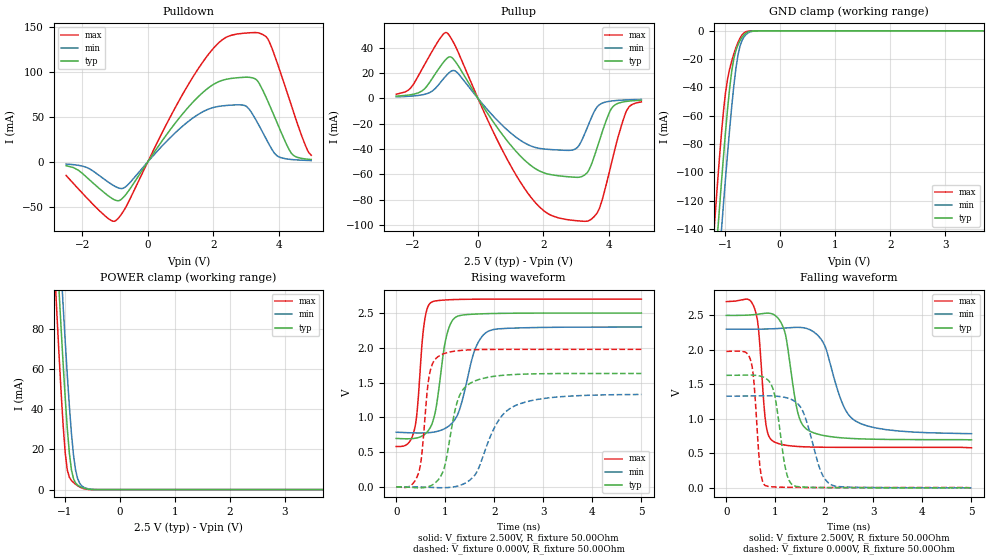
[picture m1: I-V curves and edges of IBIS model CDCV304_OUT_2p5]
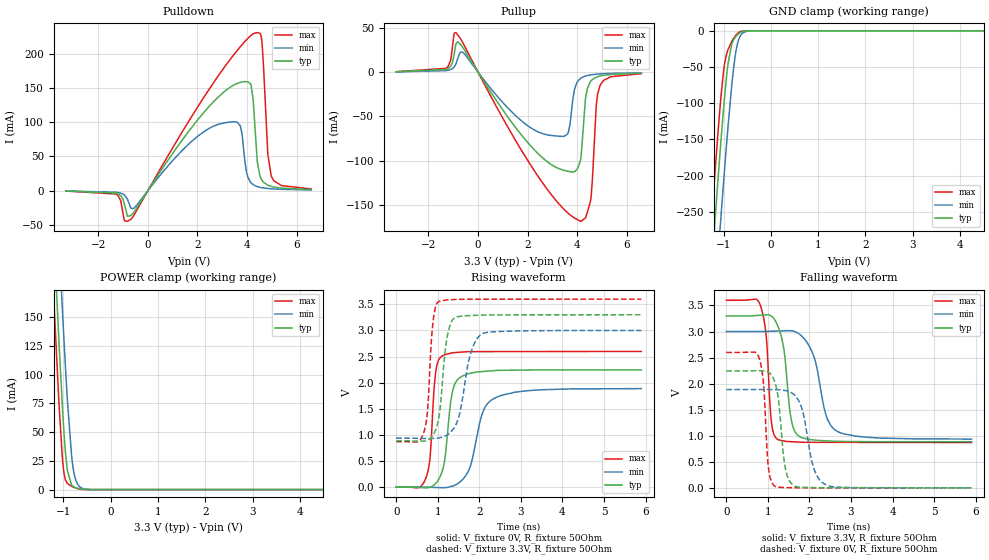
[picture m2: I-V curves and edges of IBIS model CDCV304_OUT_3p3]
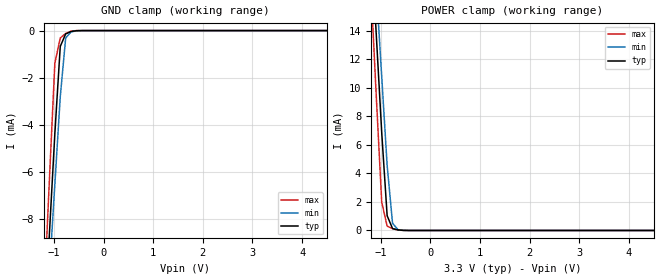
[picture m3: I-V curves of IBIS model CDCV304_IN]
|Texas Instruments Incorporated
|200-MHz General Purpose Clock Buffer, PCI-X Compliant
| Marketing part#   Voltage Range   Package-type   #pins
|CDCV304PW   2.3V - 3.6V   TSSOP   8-pin PW
|CDCV304PWG4   2.3V - 3.6V   TSSOP   8-pin PW
|CDCV304PWR   2.3V - 3.6V   TSSOP   8-pin PW
|CDCV304PWRG4   2.3V - 3.6V   TSSOP   8-pin PW
[IBIS Ver]   4.0
[File name]   cdcv304.ibs
[File Rev]   1.3
[Date]   01/30/2015
[Source]   Texas Instruments Incorporated.
   Analog-eLab, HPA
   12500 TI Blvd
   Dallas, TX -75243
   For Support e-mail: elab_ibis@list.ti.com
[Notes]   Revision History:
   Rev 1.1: 11/15/2009
   - Covers industrial temp range
   - All test data contained in this file are derived from
   hspice(tm) simulations.
   - File created by CDC Systems and Application
   Rev 1.2: 07/03/2009
   - Added CDCV304_OUT_2p5 model for 2.5V supply
   - CDCV304_OUT_2p5 model generated from TISPICED simulations
   - Non-monotonic warnings relay true buffer behavior for pullup/down
   - Added [Model Selector] to choose between 2.5V or 3.3V model.
   - Ccomp values are based on simulation setup in TISPICED,
   part uses BJT devices.
   Rev 1.3: 01/30/2015
   - Updated CDCV304_OUT_3p3 model from TISPICED simulations
   - Non-monotonic warnings relay true buffer behavior for pullup/down
[Disclaimer]
 This product is designed as an aid for customers of Texas Instruments.
 No warranties, either expressed or implied, with respect to this third
 party software (if any) or with respect to its fitness for any
 particular purpose is claimed by Texas Instruments or the author. The
 software (if any) is provided solely on an "as is" basis. The entire
 risk as to its quality and performance is with the customer
[Copyright] (C) Copyright 2009 Texas Instruments Incorporated.
   All rights reserved.
|   CDCV304PW Component
[Component]   CDCV304PW
[Manufacturer]  Texas Instruments, Inc.
[Package]   |8-pin PW TSSOP package,
|   typ   min   max
R_pkg   0.040   0.034   0.046
L_pkg   2.625nH   2.419nH   2.861nH
C_pkg   0.304pF   0.286pF   0.321pF
[Pin]   signal_name   model_name   R_pin   L_pin   C_pin
1   CLKIN   CDCV304_IN   0.12421  3.18009nH  0.51182pF
2   OE   CDCV304_IN   0.12681  2.66769nH  0.47449pF
3   1Y0   CDCV304_OUT   0.13711  2.77393nH  0.48053pF
4   GND   GND   0.08098  3.03663nH  0.54744pF
5   1Y1   CDCV304_OUT   0.12638  3.20754nH  0.51379pF
6   VDD   POWER   0.07180  2.38222nH  0.49957pF
7   1Y2   CDCV304_OUT   0.14173  2.82266nH  0.48353pF
8   1Y3   CDCV304_OUT   0.12849  3.22359nH  0.51572pF
[Model Selector] CDCV304_OUT
CDCV304_OUT_2p5   2.5V Tristate Output
CDCV304_OUT_3p3   3.3V Tristate Output
| Models and submodels in the file (3): CDCV304_OUT_2p5 (3-state), CDCV304_OUT_3p3 (3-state), CDCV304_IN (Input)
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|   Model CDCV304_OUT_2p5
[Model]   CDCV304_OUT_2p5
Model_type   3-state
Polarity   Non-Inverting
Enable   Active-High
Vmeas = 1.25V   |Vref for timing measurements.
Cref = 25pF   |load capacitance for timing spec.
Rref = 500   |500 Ohm to GND.
Vref = 0   |Timing specification test load voltage; GND
|   typ   min   max
C_comp   2.454pF   2.480pF   2.429pF
[Temperature range]   27   85   -40
[Voltage range]   2.5   2.3   2.7
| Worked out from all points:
|   slope of the pulldown table from 0 to 0.375 V, typ, clamps not added: 18.7 ohm
|   slope of the pullup table from 0 to 0.375 V, typ, clamps not added: 25.1 ohm
|   GND clamp passes 1 mA (typ) near -0.59 V on its own axis
|   POWER clamp passes 1 mA (typ) near -0.68 V on its own axis
|   falling waveform, V_fixture 2.500V, R_fixture 50.00Ohm: 20-80 % time 242ps typ, 425ps min, 133ps max; typ from 2.5 V to 0.696 V
|   rising waveform, V_fixture 2.500V, R_fixture 50.00Ohm: 20-80 % time 225ps typ, 339ps min, 143ps max; typ from 0.696 V to 2.5 V
|   rising waveform, V_fixture 0.000V, R_fixture 50.00Ohm: 20-80 % time 287ps typ, 529ps min, 159ps max; typ from 0 V to 1.63 V
|   falling waveform, V_fixture 0.000V, R_fixture 50.00Ohm: 20-80 % time 197ps typ, 325ps min, 117ps max; typ from 1.63 V to 0 V
[Pulldown]
|   Voltage   I(typ)   I(min)   I(max)
-2.5V     -4.282mA   -2.476mA   -15.1mA
-992.5mV  -42.64mA   -27.45mA   -65.62mA
-653.3mV  -35.48mA   -26.93mA   -49.07mA
703.5mV   36.48mA    27.44mA    50.95mA
1.683V    76.98mA    55.58mA    110.8mA
2.324V    90.93mA    62.24mA    136.6mA
2.965V    93.85mA    62.47mA    142.8mA
3.342V    90.38mA    44.32mA    143.3mA
3.681V    66.49mA    21.35mA    135.8mA
3.945V    44.26mA    6.972mA    111.2mA
4.397V    9.233mA    2.555mA    62.09mA
5V        2.556mA    1.432mA    7.256mA
[GND Clamp]
|   Voltage   I(typ)   I(min)   I(max)
-2.5V     -918mA     -929.6mA   -913.4mA
-1.219V   -187mA     -219.9mA   -151.3mA
-1.181V   -166.8mA   -200mA     -130.7mA
-1.143V   -146.8mA   -180.3mA   -110.7mA
-1.106V   -127.2mA   -160.9mA   -91.4mA
-1.068V   -108mA     -141.7mA   -73.33mA
-992.5mV  -71.68mA   -104.5mA   -43.83mA
-879.4mV  -28.61mA   -53.58mA   -21.34mA
-766.3mV  -9.997mA   -17.27mA   -8.262mA
-691mV    -4.522mA   -6.7mA     -2.852mA
-615.6mV  -1.453mA   -2.46mA    -549.6uA
5V        0A         0A         0A
[Pullup]
|   Voltage   I(typ)   I(min)   I(max)
-2.5V     1.763mA    1.188mA    3.233mA
-1.709V   5.877mA    2.781mA    23.11mA
-954.8mV  31.36mA    18.36mA    51.83mA
-653.3mV  27.69mA    20.84mA    39.24mA
590.5mV   -22.98mA   -17.26mA   -32.81mA
1.533V    -51.12mA   -36.53mA   -74.94mA
2.889V    -62.08mA   -40.79mA   -96.14mA
3.266V    -60.43mA   -27.98mA   -96.94mA
3.719V    -33.2mA    -4.961mA   -86.65mA
4.095V    -7.629mA   -2.04mA    -50.06mA
4.548V    -2.38mA    -1.199mA   -9.673mA
5V        -1.438mA   -849uA     -2.733mA
[POWER Clamp]
|   Voltage   I(typ)   I(min)   I(max)
-2.5V     889.6mA    895.1mA    893.4mA
-1.181V   138.6mA    167mA      107.6mA
-1.143V   118.8mA    147.5mA    87.11mA
-1.106V   99.34mA    128.4mA    67.36mA
-1.068V   80.46mA    109.6mA    48.67mA
-1.03V    62.35mA    91.33mA    31.79mA
-992.5mV  45.4mA     73.67mA    18.16mA
-954.8mV  30.26mA    56.9mA     9.72mA
-879.4mV  9.747mA    27.82mA    4.528mA
-804mV    3.293mA    9.602mA    2.651mA
-691mV    1.081mA    1.815mA    792uA
5V        0A         0A         0A
[Ramp]
R_load = 50.00Ohm
|   typ   min   max
dV/dt_r   978.461mV/286.786ps 797.286mV/528.521ps   1.187V/158.780ps
dV/dt_f   1.083V/241.882ps 909.137mV/423.978ps   1.272V/133.440ps
[Falling Waveform]
V_fixture = 2.500V
V_fixture_min = 2.300V
V_fixture_max = 2.700V
R_fixture = 50.00Ohm
|   Time   V(typ)   V(min)   V(max)
0s        2.5V       2.3V       2.7V
580ps     2.512V     2.3V       2.591V
660ps     2.519V     2.3V       2.273V
810ps     2.532V     2.303V     910.5mV
960ps     2.515V     2.306V     672.5mV
1.18ns    2.289V     2.315V     621.3mV
1.45ns    1.112V     2.326V     599.4mV
1.65ns    843.6mV    2.308V     592.7mV
2.64ns    712.2mV    965.7mV    586.2mV
5ns       695.5mV    784.7mV    580.2mV
[Rising Waveform]
V_fixture = 2.500V
V_fixture_min = 2.300V
V_fixture_max = 2.700V
R_fixture = 50.00Ohm
|   Time   V(typ)   V(min)   V(max)
0s        695.5mV    784.7mV    580.2mV
370ps     696.7mV    775.5mV    817.8mV
430ps     704.5mV    774.6mV    1.11V
570ps     749.8mV    775.4mV    2.345V
720ps     888mV      782.8mV    2.657V
1.02ns    2.152V     849.5mV    2.689V
1.23ns    2.448V     1.007V     2.695V
1.61ns    2.485V     1.983V     2.699V
1.9ns     2.492V     2.246V     2.7V
5ns       2.5V       2.3V       2.7V
[Rising Waveform]
V_fixture = 0.000V
V_fixture_min = 0.000V
V_fixture_max = 0.000V
R_fixture = 50.00Ohm
|   Time   V(typ)   V(min)   V(max)
0s        12.14uV    15.12uV    9.328uV
450ps     -14.68mV   -2.158mV   188.3mV
520ps     -14.55mV   -3.527mV   450.7mV
680ps     7.63mV     -7.739mV   1.623V
890ps     131.9mV    -13.27mV   1.889V
1.26ns    1.257V     12.05mV    1.958V
1.57ns    1.512V     140.2mV    1.972V
2.05ns    1.595V     911.9mV    1.977V
2.43ns    1.616V     1.169V     1.978V
5ns       1.631V     1.329V     1.978V
[Falling Waveform]
V_fixture = 0.000V
V_fixture_min = 0.000V
V_fixture_max = 0.000V
R_fixture = 50.00Ohm
|   Time   V(typ)   V(min)   V(max)
0s        1.631V     1.329V     1.978V
500ps     1.634V     1.332V     1.839V
560ps     1.632V     1.332V     1.553V
690ps     1.62V      1.334V     283.6mV
800ps     1.59V      1.334V     29.84mV
960ps     1.416V     1.331V     12.9mV
1.21ns    265.6mV    1.308V     7.152mV
1.37ns    32.08mV    1.265V     5.737mV
2.14ns    1.676mV    43.86mV    3.752mV
5ns       12.14uV    15.12uV    9.328uV
|   Model CDCV304_OUT_3p3
[Model]   CDCV304_OUT_3p3
Model_type   3-state
Polarity   Non-Inverting
Enable   Active-High
Vmeas = 1.5V   |Vref for timing measurements.
Cref = 15pF   |load capacitance for timing spec.
Rref = 50   |500 Ohm to GND.
Vref = 3.3   |Timing specification test load voltage; GND
|   typ   min   max
C_comp   2.8p   1.8p   3.8p
[Voltage Range]   3.3   3   3.6
[Temperature Range]   27   125   -40
[Pullup Reference]   3.3   3   3.6
[Pulldown Reference]   -0   -0   -0
[Power Clamp Reference]   3.3   3   3.6
[GND Clamp Reference]   -0   -0   -0
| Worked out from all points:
|   slope of the pulldown table from 0 to 0.495 V, typ, clamps not added: 18 ohm
|   slope of the pullup table from 0 to 0.495 V, typ, clamps not added: 22.8 ohm
|   GND clamp passes 1 mA (typ) near -0.60 V on its own axis
|   POWER clamp passes 1 mA (typ) near -0.68 V on its own axis
|   falling waveform, V_fixture 3.3V, R_fixture 50Ohm: 20-80 % time 202ps typ, 346ps min, 127ps max; typ from 3.3 V to 0.885 V
|   rising waveform, V_fixture 0V, R_fixture 50Ohm: 20-80 % time 193ps typ, 352ps min, 126ps max; typ from 0 V to 2.24 V
|   rising waveform, V_fixture 3.3V, R_fixture 50Ohm: 20-80 % time 181ps typ, 296ps min, 123ps max; typ from 0.885 V to 3.3 V
|   falling waveform, V_fixture 0V, R_fixture 50Ohm: 20-80 % time 170ps typ, 279ps min, 112ps max; typ from 2.24 V to 0 V
[Pulldown]
|   Voltage   I(typ)   I(min)   I(max)
-3.3V     -532.5uA   -429.4uA   -548.2uA
-1.29V    -3.619mA   -2.276mA   -4.881mA
-943.8mV  -19.98mA   -6.381mA   -43.94mA
-686.4mV  -36.25mA   -25.57mA   -41.88mA
1.947V    100.5mA    77.49mA    118.6mA
3.58V     156.1mA    100.2mA    203.6mA
4.165V    153.9mA    11.37mA    226.7mA
4.412V    42.4mA     6.001mA    230.7mA
4.6V      15.27mA    4.355mA    217.2mA
4.838V    8.061mA    3.213mA    53.29mA
4.976V    6.283mA    2.78mA     21.43mA
6.59V     1.714mA    1.059mA    2.521mA
[GND Clamp]
|   Voltage   I(typ)   I(min)   I(max)
-3.3V     -2.322A    -2.423A    -2.26A
-1.29V    -362.4mA   -471.1mA   -294.8mA
-1.241V   -316.7mA   -425.2mA   -249.3mA
-1.211V   -289.6mA   -397.9mA   -222.4mA
-1.063V   -158.8mA   -264.2mA   -97.15mA
-983.4mV  -95.72mA   -196mA     -48.09mA
-904.2mV  -44.97mA   -131.7mA   -25.96mA
-825mV    -18.13mA   -74.61mA   -14.72mA
-765.6mV  -10.19mA   -40.47mA   -8.301mA
-646.8mV  -2.468mA   -7.184mA   -1.172mA
-409.2mV  -10.16uA   -109.2uA   -598.7nA
6.59V     0A         0A         0A
[Pullup]
|   Voltage   I(typ)   I(min)   I(max)
-3.3V     386.2uA    255uA      448.8uA
-1.29V    3.008mA    1.667mA    4.286mA
-894.3mV  31.44mA    9.002mA    44.56mA
-597.3mV  27.08mA    21.95mA    32.33mA
3.056V    -105.9mA   -71.71mA   -141.6mA
3.63V     -111.8mA   -68.79mA   -158.8mA
4.165V    -92.99mA   -6.498mA   -168.1mA
4.343V    -28.48mA   -4.343mA   -163.7mA
4.551V    -10.15mA   -3.094mA   -142.9mA
4.769V    -5.794mA   -2.363mA   -38.76mA
4.917V    -4.449mA   -2.03mA    -15.46mA
6.59V     -1.191mA   -764uA     -1.768mA
[POWER Clamp]
|   Voltage   I(typ)   I(min)   I(max)
-3.3V     2.26A      2.342A     2.212A
-1.211V   231.7mA    322.6mA    175.8mA
-1.181V   205.3mA    296mA      149.6mA
-1.092V   129.1mA    217.9mA    75.71mA
-1.023V   75.2mA     160mA      29.73mA
-1.003V   61.41mA    144.1mA    20.6mA
-914.1mV  16.57mA    78.3mA     5.362mA
-825mV    4.071mA    29.8mA     2.929mA
-765.6mV  2.16mA     12.8mA     1.814mA
-646.8mV  654.9uA    2.29mA     376uA
-429mV    8.479uA    68.07uA    951.8nA
6.59V     0A         0A         0A
[Ramp]
R_load = 50
|   typ   min   max
dV/dt_r   1.34621/1.93407e-10   1.13168/3.51519e-10   1.55921/1.25538e-10
dV/dt_f   1.44903/2.01833e-10   1.23825/3.45663e-10   1.63784/1.27266e-10
[Falling Waveform]
V_fixture = 3.3V
V_fixture_min = 3V
V_fixture_max = 3.6V
R_fixture = 50Ohm
C_fixture = 0F
|   Time   V(typ)   V(min)   V(max)
0s        3.3V       3V         3.6V
823.7ps   3.313V     3V         3.492V
956.9ps   3.321V     3.003V     2.937V
1.098ns   3.288V     3.007V     1.185V
1.236ns   3.11V      3.01V      929.7mV
1.387ns   2.655V     3.014V     899.8mV
1.576ns   1.256V     3.013V     885.4mV
1.753ns   987.9mV    2.955V     878mV
2.626ns   893.4mV    1.106V     873.5mV
5.9ns     884.9mV    936.2mV    870.3mV
[Rising Waveform]
V_fixture = 0V
V_fixture_min = 0V
V_fixture_max = 0V
R_fixture = 50Ohm
C_fixture = 0F
|   Time   V(typ)   V(min)   V(max)
0s        170.1nV    436.6nV    30.22nV
729.2ps   -13.73mV   -2.429mV   206.2mV
809.1ps   -3.916mV   -4.43mV    526.5mV
956.9ps   75.56mV    -8.131mV   2.235V
1.118ns   331.2mV    -12.17mV   2.517V
1.361ns   1.852V     20.97mV    2.573V
1.608ns   2.133V     152.5mV    2.587V
2.103ns   2.215V     1.475V     2.595V
2.351ns   2.23V      1.695V     2.595V
5.9ns     2.244V     1.886V     2.599V
[Rising Waveform]
V_fixture = 3.3V
V_fixture_min = 3V
V_fixture_max = 3.6V
R_fixture = 50Ohm
C_fixture = 0F
|   Time   V(typ)   V(min)   V(max)
0s        884.9mV    936.2mV    870.3mV
676.6ps   881.1mV    931.4mV    1.077V
751ps     896.6mV    930.1mV    1.429V
885.2ps   998.2mV    932.6mV    3.159V
1.017ns   1.299V     939mV      3.551V
1.211ns   2.802V     989.5mV    3.584V
1.413ns   3.245V     1.162V     3.593V
1.787ns   3.286V     2.552V     3.598V
2.058ns   3.293V     2.931V     3.598V
5.9ns     3.3V       3V         3.6V
[Falling Waveform]
|Gnd
V_fixture = 0V
V_fixture_min = 0V
V_fixture_max = 0V
R_fixture = 50Ohm
C_fixture = 0F
|   Time   V(typ)   V(min)   V(max)
0s        2.244V     1.886V     2.599V
794.6ps   2.247V     1.889V     2.48V
903.1ps   2.245V     1.889V     1.92V
1.017ns   2.22V      1.889V     364.3mV
1.184ns   1.981V     1.885V     24.02mV
1.413ns   406.4mV    1.868V     5.35mV
1.64ns    38.58mV    1.782V     2.522mV
2.103ns   5.261mV    377.3mV    1.31mV
2.39ns    3.175mV    62.7mV     1.211mV
5.9ns     170.1nV    436.6nV    30.22nV
|   Model CDCV304_IN
[Model]   CDCV304_IN
Model_type   Input
Polarity   Non-Inverting
Vinl = 0.8V
Vinh = 2.0V
|   typ   min   max
C_comp   2.5pF   1.5pF   3.5pF
[Temperature range]   27   85   -40
[Voltage range]   3.3   3.0   3.6
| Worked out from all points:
|   GND clamp passes 1 mA (typ) near -0.88 V on its own axis
|   POWER clamp passes 1 mA (typ) near -0.87 V on its own axis
[GND Clamp]
|   Voltage   I(typ)   I(min)   I(max)
-3.6V     -107.1mA   -97.17mA   -122.7mA
-1.2V     -12.85mA   -13.99mA   -11.32mA
-1.091V   -8.602mA   -10.26mA   -6.296mA
-981.8mV  -4.368mA   -6.526mA   -1.382mA
-872.7mV  -672.8uA   -2.805mA   -317.4uA
-763.6mV  -139.7uA   -313.5uA   -121.8uA
-654.5mV  -39.09uA   -56.53uA   -21.47uA
-545.5mV  -4.956uA   -10.65uA   -1.188uA
-327.3mV  -13.03nA   -89.53nA   -356.9pA
7.2V      353fA      13.91pA    11.2fA
[POWER Clamp]
|   Voltage   I(typ)   I(min)   I(max)
-3.6V     171.2mA    160.5mA    186.7mA
-1.2V     20.5mA     23.21mA    17.04mA
-1.091V   13.67mA    16.99mA    9.351mA
-981.8mV  6.85mA     10.78mA    1.98mA
-872.7mV  1.033mA    4.563mA    305.4uA
-763.6mV  131.6uA    497.4uA    127.8uA
-654.5mV  40.31uA    59.57uA    30.31uA
-436.4mV  518.3nA    1.485uA    97.12nA
7.2V      -46.96pA   -908.8pA   -5.285pA
